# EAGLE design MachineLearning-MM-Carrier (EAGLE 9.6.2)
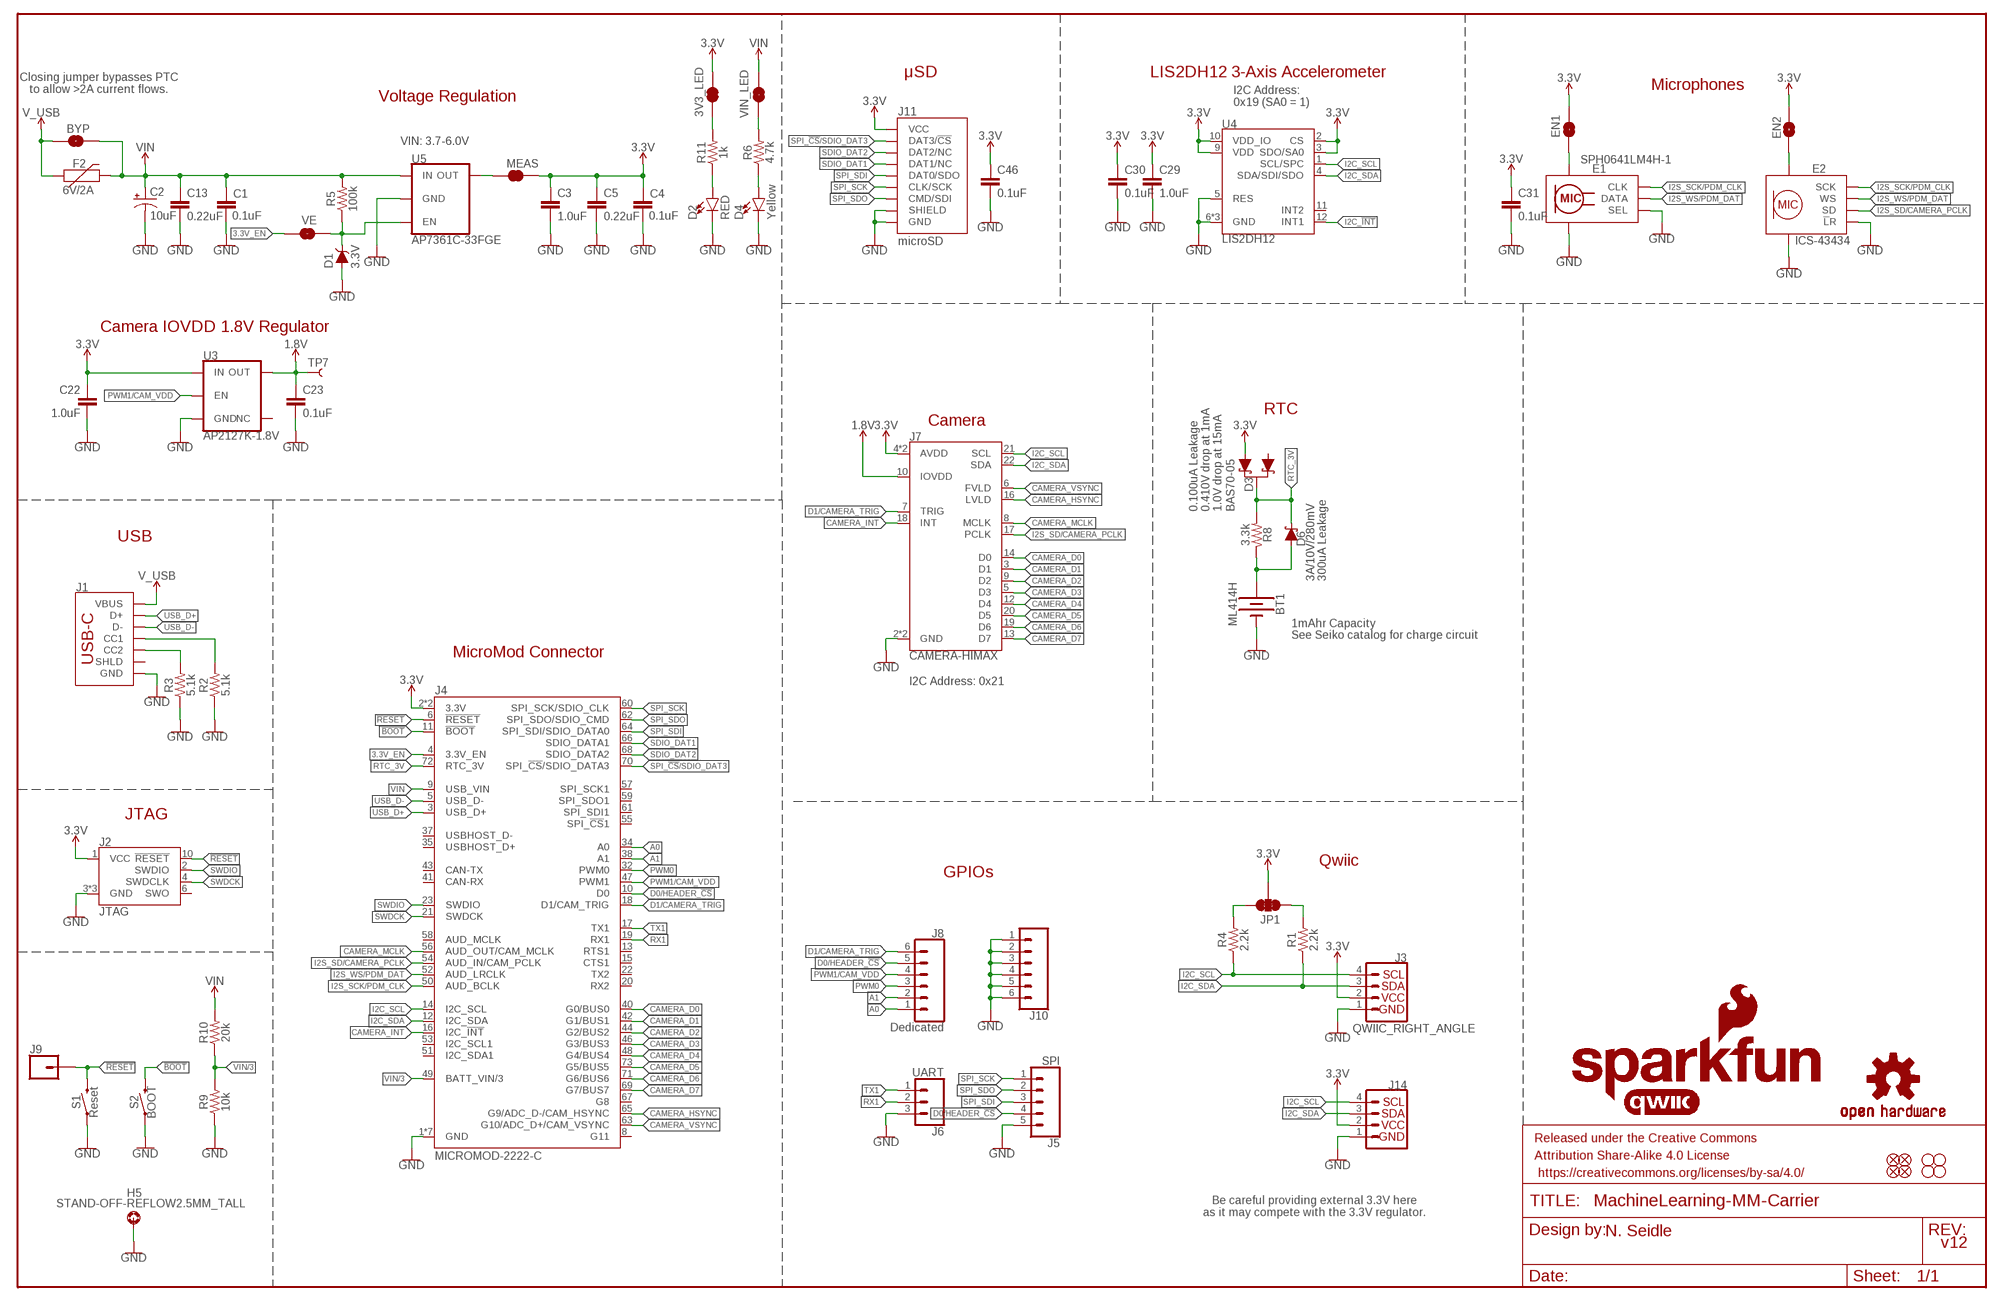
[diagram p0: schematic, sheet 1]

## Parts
3V3_LED  JUMPER-SMT_2_NC_TRACE_SILK  [SMT-JUMPER_2_NC_TRACE_SILK]
BT1  ML414H  ML414H_IV01E_BATTERY  [ML414H_IV01E]
BYP  JUMPER-SMT_2_NO_SILK  [SMT-JUMPER_2_NO_SILK]
C1  0.1uF  0.1UF-0603-25V-(+80/-20%)  [0603]
C2  10uF  10UF-POLAR-EIA3216-16V-10%(TANT)  [EIA3216]
C3  1.0uF  1.0UF-0603-16V-10%  [0603]
C4  0.1uF  0.1UF-0603-25V-(+80/-20%)  [0603]
C5  0.22uF  0.22UF-0603-25V-10%  [0603]
C13  0.22uF  0.22UF-0603-25V-10%  [0603]
C22  1.0uF  1.0UF-0603-16V-10%  [0603]
C23  0.1uF  0.1UF-0603-100V-10%  [0603]
C29  1.0uF  1.0UF-0603-16V-10%  [0603]
C30  0.1uF  0.1UF-0603-25V-(+80/-20%)  [0603]
C31  0.1uF  0.1UF-0603-25V-(+80/-20%)  [0603]
C46  0.1uF  0.1UF-0603-25V-(+80/-20%)  [0603]
D1  3.3V  DIODE-ZENER-MM3Z3V3T1G  [SOD-323]
D2  RED  LED-RED0603  [LED-0603]
D3  BAS70-05  DIODE-SCHOTTKY-DUAL  [SOT23-3]
D4  Yellow  LED-YELLOW0603  [LED-0603]
D6  3A/10V/280mV  DIODE-SCHOTTKY-BAT60A  [SOD-323]
E1  SPH0641LM4H-1  SPH0641LM4H-1_MICROPHONE  [SPH0641LM4H-1_MICROPHONE]
E2  ICS-43434  [ICS-43434]
EN1  JUMPER-SMT_2_NC_TRACE_SILK  [SMT-JUMPER_2_NC_TRACE_SILK]
EN2  JUMPER-SMT_2_NO_SILK  [SMT-JUMPER_2_NO_SILK]
F2  6V/2A  PPTC_6V2A  [1210]
FD1  FIDUCIALUFIDUCIAL  [FIDUCIAL-MICRO]
FD2  FIDUCIALUFIDUCIAL  [FIDUCIAL-MICRO]
FD3  FIDUCIALUFIDUCIAL  [FIDUCIAL-MICRO]
FD4  FIDUCIALUFIDUCIAL  [FIDUCIAL-MICRO]
FRAME1  FRAME-LEDGER  [CREATIVE_COMMONS]
H1  STAND-OFF  [STAND-OFF]
H2  STAND-OFF  [STAND-OFF]
H3  STAND-OFF  [STAND-OFF]
H4  STAND-OFF  [STAND-OFF]
H5  STAND-OFF-REFLOW2.5MM_TALL  [STAND-OFF-REFLOW-M2.5]
J1  USB_C_2-LAYER_PADS  [USB-C-16P-2LAYER-PADS]
J2  JTAG  CORTEX_JTAG_DEBUG_MINIMUM_PTH  [2X5-PTH-1.27MM]
J3  QWIIC_RIGHT_ANGLE  QWIIC_CONNECTORJS-1MM  [JST04_1MM_RA]
J4  MICROMOD-2222-C  [M.2-CONNECTOR-E]
J5  SPI  CONN_05NO_SILK  [1X05_NO_SILK]
J6  UART  CONN_031X03_NO_SILK  [1X03_NO_SILK]
J7  CAMERA-HIMAX  [FPC05024-42201]
J8  Dedicated  CONN_06NO_SILK_NO_POP  [1X06_NO_SILK]
J9  CONN_01PTH_NO_SILK_YES_STOP  [1X01_NO_SILK]
J10  CONN_06NO_SILK_NO_POP  [1X06_NO_SILK]
J11  microSD  MICRO-SD-SDIOPUSH-PUSH  [MICRO-SD-SOCKET]
J14  I2C_STANDARD_NO_SILK  [1X04_NO_SILK]
JP1  JUMPER-SMT_3_2-NC_TRACE_SILK  [SMT-JUMPER_3_2-NC_TRACE_SILK]
LOGO1  SFE_LOGO_NAME_FLAME.1_INCH  [SFE_LOGO_NAME_FLAME_.1]
LOGO2  QWIIC_LOGO_CONNECTOR  [QWIIC_5.5MM]
LOGO3  OSHW-LOGOMINI  [OSHW-LOGO-MINI]
MEAS  JUMPER-COMBO_2_NC_TRACE  [COMBO-JUMPER_2_NC_TRACE]
R1  2.2k  2.2KOHM-0603-1/10W-1%  [0603]
R2  5.1k  5.1KOHM5.1KOHM-0603-1/10W-1%  [0603]
R3  5.1k  5.1KOHM5.1KOHM-0603-1/10W-1%  [0603]
R4  2.2k  2.2KOHM-0603-1/10W-1%  [0603]
R5  100k  100KOHM-0603-1/10W-1%  [0603]
R6  4.7k  4.7KOHM-0603-1/10W-1%  [0603]
R8  3.3k  3.3KOHM-0603-1/10W-1%  [0603]
R9  10k  10KOHM-0603-1/10W-1%  [0603]
R10  20k  20KOHM-0603-1/10W-1%  [0603]
R11  1k  1KOHM-0603-1/10W-1%  [0603]
S1  Reset  MOMENTARY-SWITCH-SPST-SMD-5.2-TALL-REDUNDANT  [TACTILE_SWITCH_SMD_5.2MM]
S2  BOOT  MOMENTARY-SWITCH-SPST-SMD-5.2-TALL-REDUNDANT  [TACTILE_SWITCH_SMD_5.2MM]
TP7  TEST-POINT3X5  [PAD.03X.05]
U3  AP2127K-1.8V  V_REG_AP2127K-1.8V  [SOT23-5]
U4  LIS2DH12  [LGA-12-LISDH12]
U5  AP7361C-33FGE  AP7361C-33FGEUDFN-8  [UDFN-8]
VE  JUMPER-SMT_2_NO_SILK  [SMT-JUMPER_2_NO_SILK]
VIN_LED  JUMPER-SMT_2_NC_TRACE_SILK  [SMT-JUMPER_2_NC_TRACE_SILK]

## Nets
1.8V: C23.1 J7.10(IOVDD) TP7.P$1 U3.5(OUT)
3.3V: 3V3_LED.2 C3.1 C4.1 C5.1 C22.1 C29.1 C30.1 C31.1 C46.1 D3.2(A1) EN1.2 EN2.2 J2.1(VCC) J3.2 J4.2(3.3V) J4.74(3.3V) J7.4(AVDD) J7.11(AVDD) J11.VCC J14.2 JP1.2 MEAS.2 MEAS.4 U3.1(IN) U4.2(CS) U4.3(SDO/SA0) U4.9(VDD) U4.10(VDD_IO)
3.3V_EN: J4.4(3.3V_EN) VE.1
!BOOT!: J4.11(!BOOT!) S2.3 S2.4
!RESET!: J2.10(!RESET) J4.6(!RESET!) J9.1 S1.3 S1.4
A0: J4.34(A0) J8.1
A1: J4.38(A1) J8.2
CAMERA_D0: J4.40(G0/BUS0) J7.14(D0)
CAMERA_D1: J4.42(G1/BUS1) J7.3(D1)
CAMERA_D2: J4.44(G2/BUS2) J7.9(D2)
CAMERA_D3: J4.46(G3/BUS3) J7.5(D3)
CAMERA_D4: J4.48(G4/BUS4) J7.12(D4)
CAMERA_D5: J4.73(G5/BUS5) J7.20(D5)
CAMERA_D6: J4.71(G6/BUS6) J7.19(D6)
CAMERA_D7: J4.69(G7/BUS7) J7.13(D7)
CAMERA_HSYNC: J4.65(G9/ADC_D-/CAM_HSYNC) J7.16(LVLD)
CAMERA_INT: J4.16(I2C_!INT!) J7.18(INT)
CAMERA_MCLK: J4.56(AUD_OUT/CAM_MCLK) J7.8(MCLK)
CAMERA_VSYNC: J4.63(G10/ADC_D+/CAM_VSYNC) J7.6(FVLD)
D0/HEADER_!CS!: J4.10(D0) J5.4 J8.5
D1/CAMERA_TRIG: J4.18(D1/CAM_TRIG) J7.7(TRIG) J8.6
GND: BT1.- C1.2 C2.- C3.2 C4.2 C5.2 C13.2 C22.2 C23.2 C29.2 C30.2 C31.2 C46.2 D1.A D2.C D4.C E1.2(SEL) E1.3(GND) E1.6(GND) E1.7(GND) E1.8(GND) E2.2(!L!R) E2.3(GND) E2.7(GND) E2.8(GND) E2.9(GND) H5.1 J1.GND J1.GND2(GND) J2.3(GND) J2.5(GND) J2.9(GND) J3.1 J4.1(GND) J4.7(GND) J4.33(GND) J4.36(GND) J4.39(GND) J4.45(GND) J4.75(GND) J5.5 J6.3 J7.2(GND) J7.15(GND) J10.1 J10.2 J10.3 J10.4 J10.5 J10.6 J11.CD1(SHIELD) J11.GND J11.GND1(GND) J11.GND3(GND) J14.1 R2.1 R3.1 R9.1 S1.1 S1.2 S2.1 S2.2 U3.2(GND) U4.5(RES) U4.6(GND) U4.7(GND) U4.8(GND) U5.4(GND) U5.EP(GND)
I2C_!INT!: U4.12(INT1)
I2C_SCL: J3.4 J4.14(I2C_SCL) J7.21(SCL) J14.4 R4.1 U4.1(SCL/SPC)
I2C_SDA: J3.3 J4.12(I2C_SDA) J7.22(SDA) J14.3 R1.1 U4.4(SDA/SDI/SDO)
I2S_SCK/PDM_CLK: E1.4(CLK) E2.4(SCK) J4.50(AUD_BCLK)
I2S_SD/CAMERA_PCLK: E2.6(SD) J4.54(AUD_IN/CAM_PCLK) J7.17(PCLK)
I2S_WS/PDM_DAT: E1.1(DATA) E2.1(WS) J4.52(AUD_LRCLK)
N$1: R6.2 VIN_LED.1
N$2: JP1.3 R4.2
N$3: JP1.1 R1.2
N$4: E1.5(VDD) EN1.1
N$5: E2.5(VDD) EN2.1
N$6: 3V3_LED.1 R11.2
N$7: D2.A R11.1
N$8: D4.A R6.1
N$10: J1.A5(CC1) R2.2
N$11: J1.B5(CC2) R3.2
N$12: D1.C R5.1 U5.5(EN) VE.2
N$14: BT1.+ D6.A R8.1
PWM0: J4.32(PWM0) J8.3
PWM1/CAM_VDD: J4.47(PWM1) J8.4 U3.3(EN)
RTC_3V: D3.3(C) D6.C J4.72(RTC_3V) R8.2
RX1: J4.19(RX1) J6.2
SDIO_DAT1: J4.66(SDIO_DATA1) J11.DAT1(DAT1/NC)
SDIO_DAT2: J4.68(SDIO_DATA2) J11.DAT2(DAT2/NC)
SPI_!CS!/SDIO_DAT3: J4.70(SPI_!CS!/SDIO_DATA3) J11.CS/DAT3(DAT3/!CS!)
SPI_SCK: J4.60(SPI_SCK/SDIO_CLK) J5.1 J11.SCLK(CLK/SCK)
SPI_SDI: J4.64(SPI_SDI/SDIO_DATA0) J5.3 J11.DO/DAT0(DAT0/SDO)
SPI_SDO: J4.62(SPI_SDO/SDIO_CMD) J5.2 J11.DI/CMD(CMD/SDI)
SWDCK: J2.4(SWDCLK) J4.21(SWDCK)
SWDIO: J2.2(SWDIO) J4.23(SWDIO)
TX1: J4.17(TX1) J6.1
USB_D+: J1.A6(D+) J1.B6(D+) J4.3(USB_D+)
USB_D-: J1.A7(D-) J1.B7(D-) J4.5(USB_D-)
V_USB: BYP.1 F2.1 J1.VBUS1(VBUS) J1.VBUS2(VBUS)
VIN: BYP.2 C1.1 C2.+ C13.1 F2.2 J4.9(USB_VIN) R5.2 R10.2 U5.8(IN) VIN_LED.2
VIN/3: J4.49(BATT_VIN/3) R9.2 R10.1
VREG_3.3V: MEAS.1 MEAS.3 U5.1(OUT)
Unconnected: D3.1(A) J1.SHLD1(SHLD) J1.SHLD2(SHLD) J1.SHLD3(SHLD) J1.SHLD4(SHLD) J2.6(SWO) J4.8(G11) J4.13(RTS1) J4.15(CTS1) J4.20(RX2) J4.22(TX2) J4.35(USBHOST_D+) J4.37(USBHOST_D-) J4.41(CAN-RX) J4.43(CAN-TX) J4.51(I2C_SDA1) J4.53(I2C_SCL1) J4.55(SPI_!CS!1) J4.57(SPI_SCK1) J4.58(AUD_MCLK) J4.59(SPI_SDO1) J4.61(SPI_SDI1) J4.67(G8) J7.MNT1 J7.MNT2 U3.4(NC) U4.11(INT2)

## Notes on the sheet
- μSD | LIS2DH12 3-Axis Accelerometer
- Closing jumper bypasses PTC
  to allow >2A current flows.
- Microphones
- Voltage Regulation
- I2C Address:
  0x19 (SA0 = 1)
- VIN: 3.7-6.0V
- Camera IOVDD 1.8V Regulator
- RTC
- Camera
- 0.100uA Leakage
  0.410V drop at 1mA
  1.0V drop at 15mA
- USB
- 300uA Leakage
- 1mAhr Capacity
- See Seiko catalog for charge circuit
- MicroMod Connector
- I2C Address: 0x21
- JTAG
- Qwiic
- GPIOs
- Be careful providing external 3.3V here
  as it may compete with the 3.3V regulator.
- N. Seidle
- v12

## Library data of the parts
3V3_LED EN1 VIN_LED = SparkFun-Jumpers:JUMPER-SMT_2_NC_TRACE: Normally closed trace jumper
BT1 = SparkFun-Batteries:ML414H_IV01E_BATTERY: SEIKO ML414H-IV01E Reflowable Lithium Battery; PROD_ID: BATT-14267
BYP EN2 VE = SparkFun-Jumpers:JUMPER-SMT_2_NO: Normally open jumper
C1 C4 C30 C31 C46 = SparkFun-Capacitors:0.1UF: 0.1µF ceramic capacitors; PROD_ID: CAP-00810
C2 = SparkFun-Capacitors:10UF-POLAR: 10.0µF polarized capacitors; PROD_ID: CAP-00811
C3 C22 C29 = SparkFun-Capacitors:1.0UF: 1µF ceramic capacitors; PROD_ID: CAP-00868
C5 C13 = SparkFun-Capacitors:0.22UF: 0.22µF ceramic capacitors; PROD_ID: CAP-07822
C23 = SparkFun-Capacitors:0.1UF: 0.1µF ceramic capacitors; PROD_ID: CAP-08390
D1 = SparkFun-DiscreteSemi:DIODE-ZENER: Zener Diode; PROD_ID: DIO-11284
D2 = SparkFun-LED:LED-RED: Red SMD LED; PROD_ID: DIO-00819
D3 = SparkFun-DiscreteSemi:DIODE-SCHOTTKY-DUAL: Diodes Incorporated - BAS70-05 Dual Schottky Diode Two Schottky Diodes in a single SOT-23 package. Low reverse current (100 nA) Vf: Datasheet referenced for footprint; PROD_ID: DIO-14829
D4 = SparkFun-LED:LED-YELLOW: Yellow SMD LED; PROD_ID: DIO-09003
D6 = SparkFun-DiscreteSemi:DIODE-SCHOTTKY: Schottky diode; PROD_ID: DIO-14072
E1 = SparkFun-Sensors:SPH0641LM4H-1_MICROPHONE: SPH0641LM4H-1 Microphone A miniature, high-performance, low power, bottom port silicon digital microphone with a single bit PDM output.; PROD_ID: IC-14361
E2 = Teensy:ICS-43434; PROD_ID: COMP-14898
F2 = SparkFun-Fuses:PPTC: Resettable Fuse PPTC; PROD_ID: RES-14313
FD1-FD4 = SparkFun-Aesthetics:FIDUCIAL: Fiducial Alignment Points
FRAME1 = SparkFun-Aesthetics:FRAME-LEDGER: Schematic Frame - Ledger
H1-H4 = SparkFun-Hardware:STAND-OFF: Stand Off
H5 = SparkFun-Hardware:STAND-OFF-REFLOW: Stand Off Reflow Compatible; PROD_ID: HW-14899
J1 = SparkFun-Connectors:USB_C: USB Type C 16Pin Connector Super Speed pins not available on the 16-pin purely SMD connector so this part is best for USB 2.0 implementations. D1 and D2 are tied together enabling D+/- no matter which way the cable is plugged into the connector. The two channel configuration pins (CC1/2) are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; PROD_ID: CONN-14122
J2 = SparkFun-Connectors:CORTEX_JTAG_DEBUG_MINIMUM: Cortex Debug Connector - 10 pin Supports JTAG debug, Serial Wire debug, and Serial Wire Viewer. PTH and SMD connector options available. General Connector Information Products: PTH Connector -via Digi-Key SparkFun PSoc SparkFun T
J3 = SparkFun-Connectors:QWIIC_CONNECTOR: SparkFun I2C Standard Qwiic Connector An SMD 1mm pitch JST connector makes it easy and quick (get it? Qwiic?) to connect I2C devices to each other. The Qwiic system enables fast and solderless connection between popular platforms and various sensors and actuators. We carry 200mm, 100mm, 50mm, and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; PROD_ID: CONN-13694
J4 = SparkFun-MicroMod:MICROMOD: MicroMod Connector Description: A card edge connector and mating PCB connector to allow various MicroMod Processor Boards to be coupled with various carrier boards of different capabilities. Based on the M.2 standard.; PROD_ID: CONN-14877
J5 = SparkFun-Connectors:CONN_05: Multi connection point. Often used as Generic Header-pin footprint for 0.1 inch spaced/style header connections On any of the 0.1 inch spaced packages, you can populate with these: Break Away Headers - Straight (PRT-00116) Break Away Male Headers - Right Angle (PRT-00553) Female Headers (PRT-00115)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
J6 = SparkFun-Connectors:CONN_03: Multi connection point. Often used as Generic Header-pin footprint for 0.1 inch spaced/style header connections On any of the 0.1 inch spaced packages, you can populate with these: Break Away Headers - Straight (PRT-00116) Break Away Male Headers - Right Angle (PRT-00553) Female Headers (PRT-00115)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
J7 = SparkFun-Connectors:CAMERA-HIMAX
J8 J10 = SparkFun-Connectors:CONN_06: Multi connection point. Often used as Generic Header-pin footprint for 0.1 inch spaced/style header connections On any of the 0.1 inch spaced packages, you can populate with these: Break Away Headers - Straight (PRT-00116) Break Away Male Headers - Right Angle (PRT-00553) Female Headers (PRT-00115)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
J9 = SparkFun-Connectors:CONN_01: Single connection point. Often used as Generic Header-pin footprint for 0.1 inch spaced/style header connections
J11 = SparkFun-Connectors:MICRO-SD-SDIO: microSD Socket for Transflash Push-push type µSD socket. tDoc lines correctly indicate media card edge positions when inserting (unlocked, locked, depressed). NOTE: CD1 and CD2 are connected internally, and the default detect state of the socket is detect pin to ground. SparkFun Products: WAV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; PROD_ID: CONN-07820
J14 = SparkFun-Connectors:I2C_STANDARD: SparkFun I2C Standard Pinout Header SparkFun has standardized on a pinout for all I2C based sensor breakouts. This pinout allows I2C boards to be plugged directly into the headers on Arduino Uno compatible boards, and to be daisy chained easily. Example SparkFun Products: SparkFun Atmospheric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
JP1 = SparkFun-Jumpers:JUMPER-SMT_3_2-NC_TRACE: Normally closed trace jumper (2 of 2 connections) This jumper has a trace between all three pads so they are normally closed (NC). Use a razor knife to open the connection(s). For best results follow the IPC guidelines for cutting traces: Cutout at least 0.063 mm (0.005 in). Remove all loose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
LOGO1 = SparkFun-Aesthetics:SFE_LOGO_NAME_FLAME: SparkFun Font Logo w/ Flame
LOGO2 = SparkFun-Aesthetics:QWIIC_LOGO: Qwiic Logos for placement on schematic and PCB. The 5.5mm silk logo is best for placing next to Qwiic connector.
LOGO3 = SparkFun-Aesthetics:OSHW-LOGO: Open-Source Hardware (OSHW) Logo
MEAS = SparkFun-Jumpers:JUMPER-COMBO_2_NC_TRACE
R1 R4 = SparkFun-Resistors:2.2KOHM: 2.2kΩ resistor; PROD_ID: RES-08272
R2 R3 = SparkFun-Resistors:5.1KOHM; PROD_ID: RES-12083
R5 = SparkFun-Resistors:100KOHM: 100kΩ resistor; PROD_ID: RES-07828
R6 = SparkFun-Resistors:4.7KOHM: 4.7kΩ resistor; PROD_ID: RES-07857
R8 = SparkFun-Resistors:3.3KOHM: 3.3kΩ resistor; PROD_ID: RES-07851
R9 = SparkFun-Resistors:10KOHM: 10kΩ resistor; PROD_ID: RES-00824
R10 = SparkFun-Resistors:20KOHM: 20kΩ resistor; PROD_ID: RES-09383
R11 = SparkFun-Resistors:1KOHM: 1kΩ resistor; PROD_ID: RES-07856
S1 S2 = SparkFun-Switches:MOMENTARY-SWITCH-SPST: Momentary Switch (Pushbutton) - SPST; PROD_ID: SWCH-14139
TP7 = SparkFun-Connectors:TEST-POINT: SparkFun Test Points
U3 = SparkFun-IC-Power:V_REG_AP2127: AP2127 - 300mA CMOS LDO Regulator w/ Enable The AP2127 is CMOS process low dropout linear regulator with enable function, the regulator delivers a guaranteed 300mA (min.) continuous load current. Features Output Voltage Accuracy: ±1.5% Output Current: 300mA (Min.) Foldback Short Current Protection: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; PROD_ID: VREG-14239
U4 = SparkFun-Sensors:LIS2DH12; DIGIKEY: 497-14851-2-ND; PROD_ID: IC-14229
U5 = SparkFun-IC-Power:AP7361C-33FGE: AP7361C 3.3V LDO Regulator; PROD_ID: VREG-14094

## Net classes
0 default: width 0 mm, drill 0 mm
1 power: width 0.762 mm

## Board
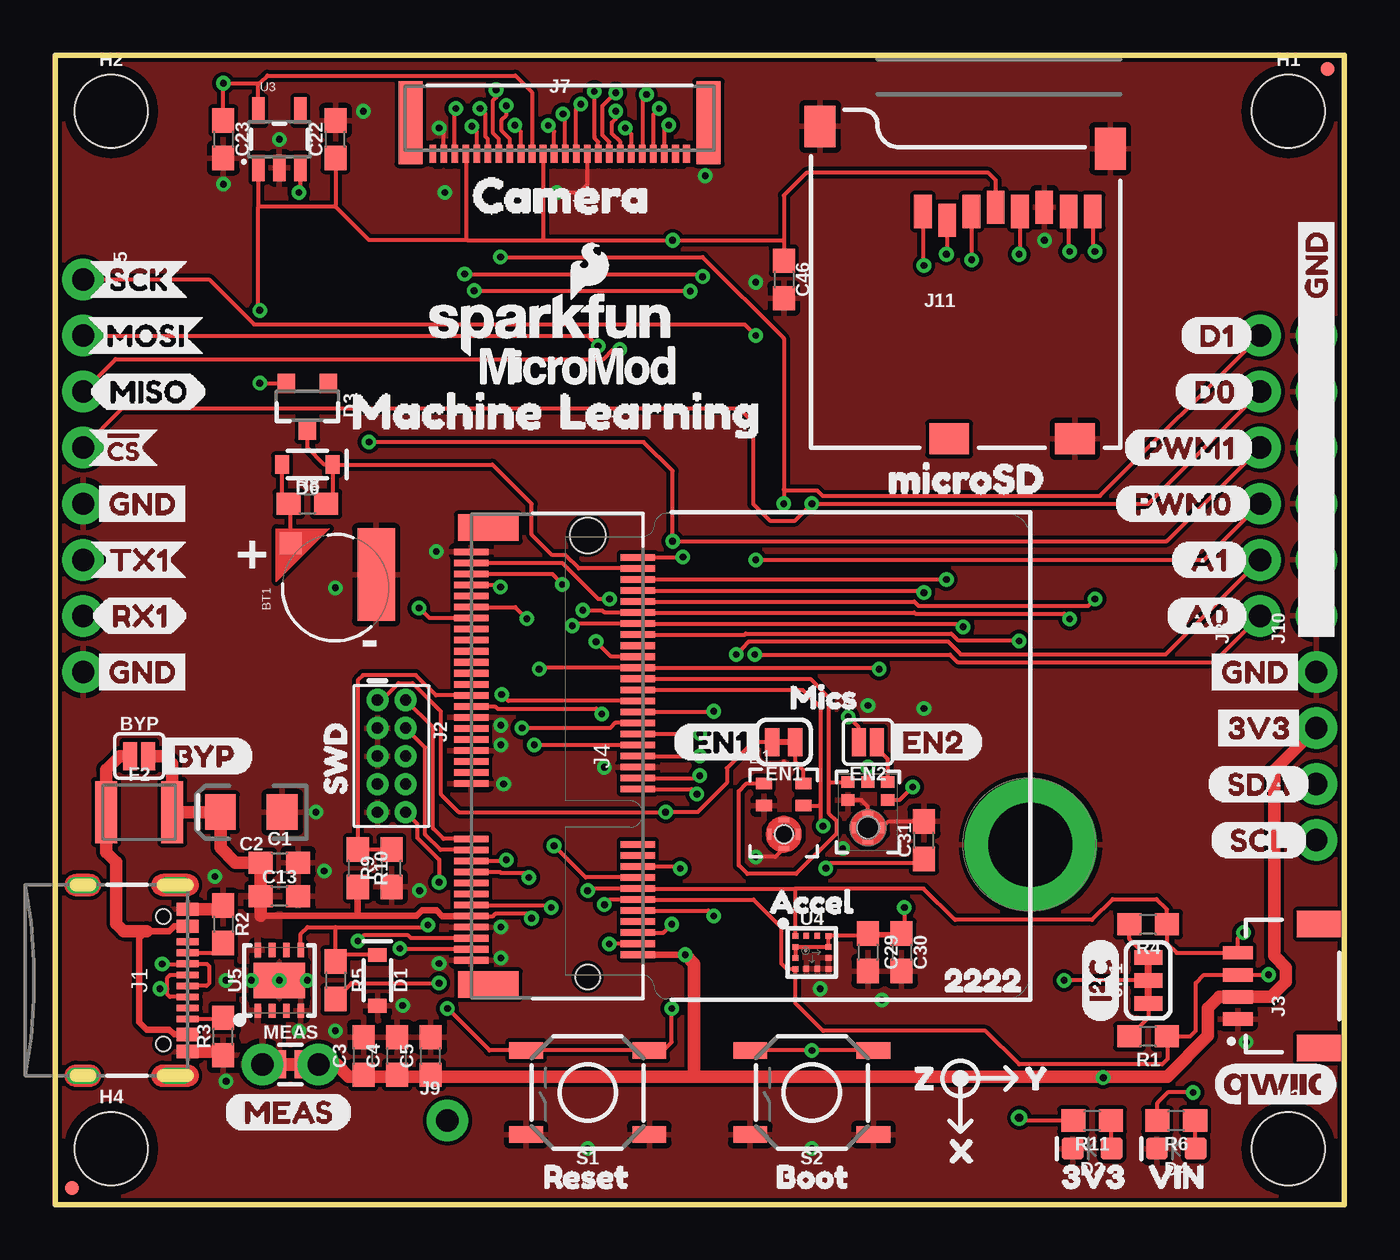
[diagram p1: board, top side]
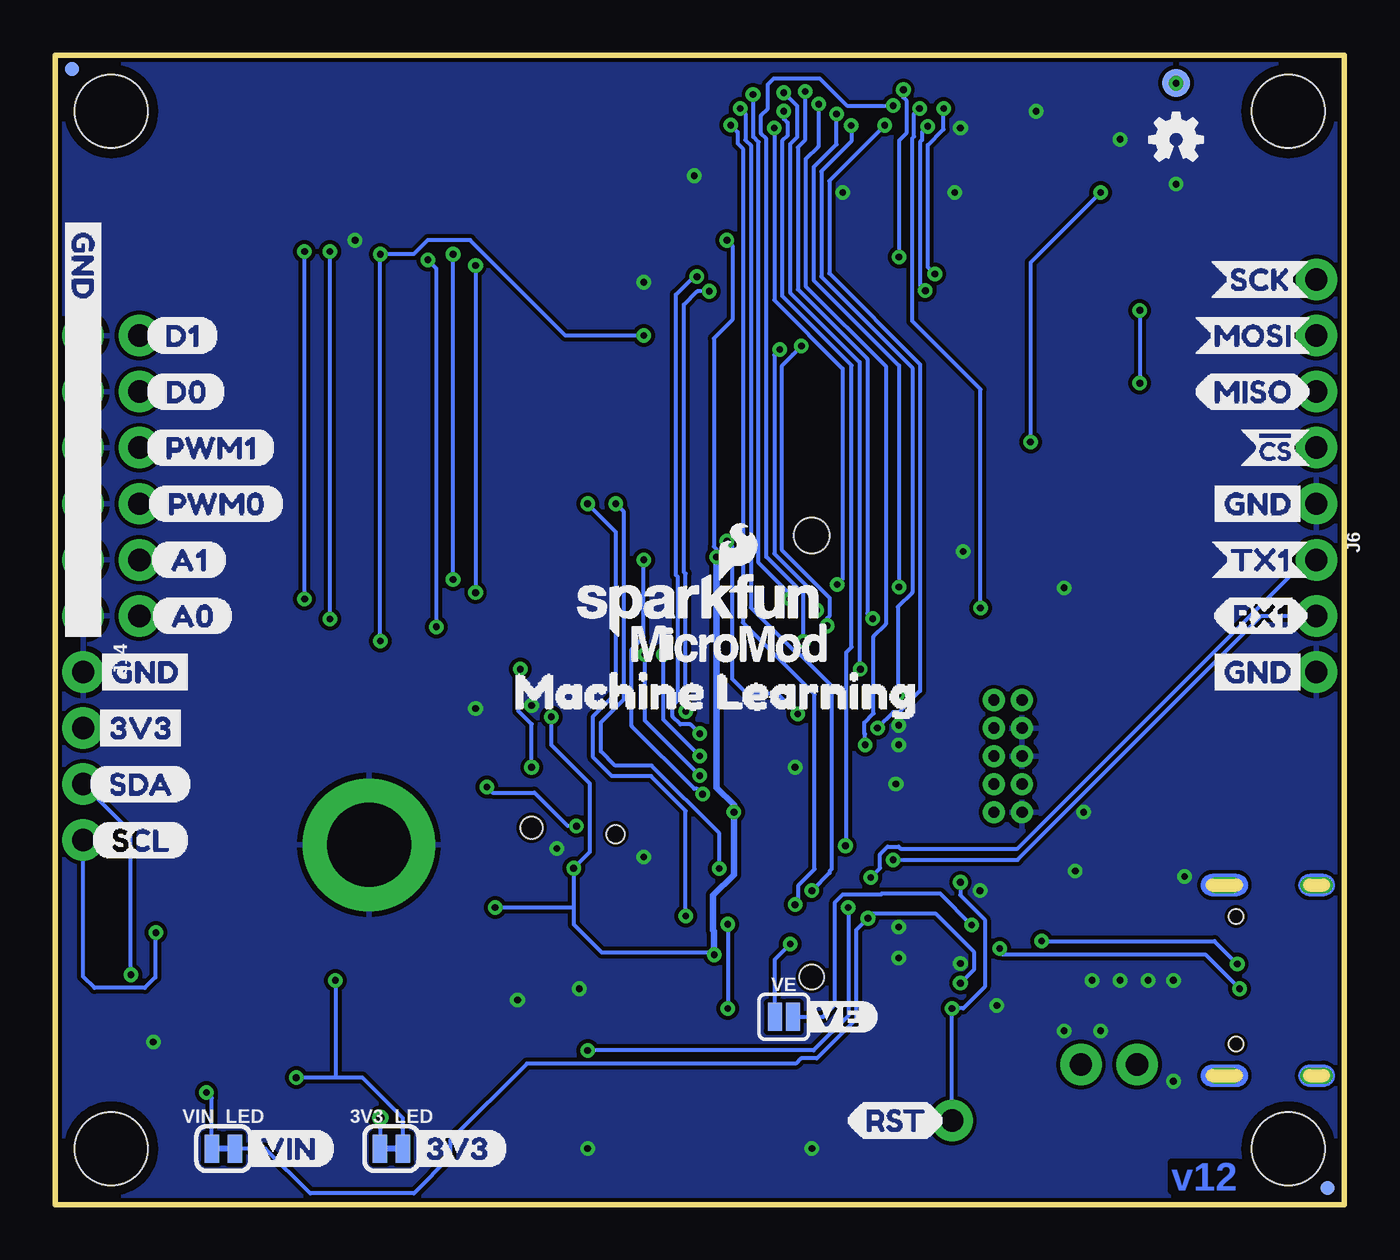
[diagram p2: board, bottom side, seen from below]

Size 58.42 x 52.07 mm. Coordinates in mm from the lower left corner, seen from the top.
Outline: 0,0 0,52.07 58.42,52.07 58.42,0 0,0
Copper layers (1*16): Top 0.035mm / dielectric 1.5mm / Bottom 0.035mm
Design rules "SparkFun-2-layer-TIGHT *": minimum track width 7mil, minimum drill 12mil, track to track 7mil, track to pad 7mil, pad to pad 7mil, via to via 7mil, smd to smd 7mil, copper to edge 7mil, drill to drill 7mil, minimum pad ring 7mil, minimum via ring 7mil, stop-mask expansion 4mil, vias tented up to drill 25mil, thermal gap 10mil

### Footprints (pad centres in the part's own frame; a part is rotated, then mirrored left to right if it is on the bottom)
SMT-JUMPER_2_NC_TRACE_SILK = smd 0.66 x 1.27: 1 -0.521,0; 2 0.521,0
ML414H_IV01E = smd 1 x 1: + 2.022,2.032 | smd 4.2 x 1.7: - 0.6,-1.85
SMT-JUMPER_2_NO_SILK = smd 0.635 x 1.27: 1 -0.406,0; 2 0.406,0
0603 = smd 1.1 x 1: 1 -0.85,0; 2 0.85,0
EIA3216 = smd 1.4 x 1.6: + 1.4,0; - -1.4,0
SOD-323 = smd 0.63 x 0.83: A 1.15,0; C -1.15,0
LED-0603 = smd 1 x 1: A -0.877,0; C 0.877,0
SOT23-3 = smd 0.8 x 0.9: 1 -0.95,-1; 2 0.95,-1; 3 0,1.1
SPH0641LM4H-1_MICROPHONE = smd 0.725 x 0.522: 1 -0.9,1.3; 2 -0.9,0.3; 4 0.9,0.3; 5 0.9,1.3 | smd 0.5 x 0.2: 3 0,-1.65; 8 0,-0.35 | smd 0.2 x 0.5: 6 -0.65,-1; 7 0.65,-1 | hole 0.8: 0,-1
ICS-43434 = smd 0.522 x 0.6: 1 -1.364,-0.9; 2 -0.542,-0.9; 4 -0.542,0.9; 5 -1.364,0.9; 6 -1.364,0 | smd 0.2 x 0.5: 3 1.36,0; 8 0.06,0 | smd 0.5 x 0.2: 7 0.71,0.65; 9 0.71,-0.65 | hole 1: 0.71,0
1210 = smd 1 x 2.8: 1 -1.5,0; 2 1.5,0
FIDUCIAL-MICRO = smd 0.635 x 0.635: 1 0,0
STAND-OFF = hole 3.302: 0,0
STAND-OFF-REFLOW-M2.5 = drill 3.8 pad 6: 1 0,0
USB-C-16P-2LAYER-PADS = smd 0.3 x 1: A5 -1.25,-0.34; A6 -0.25,-0.34; A7 0.25,-0.34; A8 1.25,-0.34; B5 1.75,-0.34; B6 0.75,-0.34; B7 -0.75,-0.34; B8 -1.75,-0.34 | smd 0.6 x 1: GND -3.225,-0.34; GND2 3.225,-0.34; VBUS1 -2.45,-0.34; VBUS2 2.45,-0.34 | drill 0.4 pad 0.6 long: SHLD1 -4.318,-0.915; SHLD2 4.318,-0.915; SHLD3 -4.318,-5.095; SHLD4 4.318,-5.095 | hole 0.65: -2.89,-1.445; 2.89,-1.445
2X5-PTH-1.27MM = drill 0.508 pad 1: 1 -2.54,-0.635; 2 -2.54,0.635; 3 -1.27,-0.635; 4 -1.27,0.635; 5 0,-0.635; 6 0,0.635; 7 1.27,-0.635; 8 1.27,0.635; 9 2.54,-0.635; 10 2.54,0.635
JST04_1MM_RA = smd 0.6 x 1.35: 1 -1.5,0; 2 -0.5,0; 3 0.5,0; 4 1.5,0 | smd 1.2 x 2: NC1 2.8,-3.675; NC2 -2.8,-3.675
M.2-CONNECTOR-E = smd 0.3 x 1.55: 1 9.25,-5.275; 2 9,2.275; 3 8.75,-5.275; 4 8.5,2.275; 5 8.25,-5.275; 6 8,2.275; 7 7.75,-5.275; 8 7.5,2.275; 9 7.25,-5.275; 10 7,2.275; 11 6.75,-5.275; 12 6.5,2.275; 13 6.25,-5.275; 14 6,2.275; 15 5.75,-5.275; 16 5.5,2.275; 17 5.25,-5.275; 18 5,2.275; 19 4.75,-5.275; 20 4.5,2.275; 21 4.25,-5.275; 22 4,2.275; 23 3.75,-5.275; 32 1.5,2.275; 33 1.25,-5.275; 34 1,2.275; 35 0.75,-5.275; 36 0.5,2.275; 37 0.25,-5.275; 38 0,2.275; 39 -0.25,-5.275; 40 -0.5,2.275; 41 -0.75,-5.275; 42 -1,2.275; 43 -1.25,-5.275; 44 -1.5,2.275; 45 -1.75,-5.275; 46 -2,2.275; 47 -2.25,-5.275; 48 -2.5,2.275; 49 -2.75,-5.275; 50 -3,2.275; 51 -3.25,-5.275; 52 -3.5,2.275; 53 -3.75,-5.275; 54 -4,2.275; 55 -4.25,-5.275; 56 -4.5,2.275; 57 -4.75,-5.275; 58 -5,2.275; 59 -5.25,-5.275; 60 -5.5,2.275; 61 -5.75,-5.275; 62 -6,2.275; 63 -6.25,-5.275; 64 -6.5,2.275; 65 -6.75,-5.275; 66 -7,2.275; 67 -7.25,-5.275; 68 -7.5,2.275; 69 -7.75,-5.275; 70 -8,2.275; 71 -8.25,-5.275; 72 -8.5,2.275; 73 -8.75,-5.275; 74 -9,2.275; 75 -9.25,-5.275 | smd 1.2 x 2.75: A1 10.35,-4.5; A2 -10.35,-4.5 | hole 1.1: 10,0 | hole 1.6: -10,0
1X05_NO_SILK = drill 1.016 pad 1.88: 1 0,0; 2 2.54,0; 3 5.08,0; 4 7.62,0; 5 10.16,0
1X03_NO_SILK = drill 1.016 pad 1.88: 1 0,0; 2 2.54,0; 3 5.08,0
FPC05024-42201 = smd 0.3 x 0.8: 1 5.75,0.4; 2 5.25,0.4; 3 4.75,0.4; 4 4.25,0.4; 5 3.75,0.4; 6 3.25,0.4; 7 2.75,0.4; 8 2.25,0.4; 9 1.75,0.4; 10 1.25,0.4; 11 0.75,0.4; 12 0.25,0.4; 13 -0.25,0.4; 14 -0.75,0.4; 15 -1.25,0.4; 16 -1.75,0.4; 17 -2.25,0.4; 18 -2.75,0.4; 19 -3.25,0.4; 20 -3.75,0.4; 21 -4.25,0.4; 22 -4.75,0.4; 23 -5.25,0.4; 24 -5.75,0.4 | smd 1.1 x 3.75: MNT1 -6.75,-1; MNT2 6.75,-1
1X06_NO_SILK = drill 1.016 pad 1.88: 1 0,0; 2 2.54,0; 3 5.08,0; 4 7.62,0; 5 10.16,0; 6 12.7,0
1X01_NO_SILK = drill 1.016 pad 1.88: 1 0,0
MICRO-SD-SOCKET = smd 1.8 x 1.4: CD1 -2.05,0.4; CD2 -7.75,0.4 | smd 0.8 x 1.5: CS/DAT3 -7.84,10.3; DAT1 -1.24,10.7; DAT2 -8.94,10.7; DI/CMD -6.74,10.7; DO/DAT0 -2.34,10.7; GND -3.44,10.9; SCLK -4.54,10.7; VCC -5.64,10.9 | smd 1.4 x 1.9: GND1 -13.6,14.55; GND3 -0.45,13.55
1X04_NO_SILK = drill 1.016 pad 1.88: 1 0,0; 2 2.54,0; 3 5.08,0; 4 7.62,0
SMT-JUMPER_3_2-NC_TRACE_SILK = smd 0.66 x 1.27: 1 -1.041,0; 2 0,0; 3 1.041,0
COMBO-JUMPER_2_NC_TRACE = smd 0.635 x 1.27: 1 -0.508,0; 2 0.508,0 | drill 1.016 pad 1.88: 3 -1.27,0; 4 1.27,0
TACTILE_SWITCH_SMD_5.2MM = smd 1.524 x 0.762: 1 -2.794,1.905; 2 2.794,1.905; 3 -2.794,-1.905; 4 2.794,-1.905
PAD.03X.05 = smd 1.27 x 1.27: P$1 0,0
SOT23-5 = smd 0.55 x 1.2: 1 -0.95,-1.3; 2 0,-1.3; 3 0.95,-1.3; 4 0.95,1.3; 5 -0.95,1.3
LGA-12-LISDH12 = smd 0.275 x 0.25: 1 -0.75,0.75; 2 -0.75,0.25; 3 -0.75,-0.25; 4 -0.75,-0.75; 7 0.75,-0.75; 8 0.75,-0.25; 9 0.75,0.25; 10 0.75,0.75 | smd 0.25 x 0.275: 5 -0.25,-0.75; 6 0.25,-0.75; 11 0.25,0.75; 12 -0.25,0.75
UDFN-8 = smd 0.3 x 0.65: 1 -0.975,-1.375; 2 -0.325,-1.375; 3 0.325,-1.375; 4 0.975,-1.375; 5 0.975,1.375; 6 0.325,1.375; 7 -0.325,1.375; 8 -0.975,1.375 | smd 2.35 x 1.6: EP 0,0

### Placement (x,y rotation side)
3V3_LED  43.18,2.54 0 bottom
BT1  12.7,27.94 90 top
BYP  3.81,20.32 0 top
C1  10.16,15.49 0 top
C2  8.89,17.78 180 top
C3  13.97,6.73 90 top
C4  15.49,6.73 90 top
C5  17.02,6.73 90 top
C13  10.16,13.97 0 top
C22  12.7,48.26 90 top
C23  7.62,48.26 270 top
C29  36.83,11.43 270 top
C30  38.35,11.43 270 top
C31  39.37,16.51 90 top
C46  33.02,41.91 270 top
D1  14.61,10.16 270 top
D2  46.99,2.54 180 top
D3  11.43,36.2 180 top
D4  50.8,2.54 180 top
D6  11.43,33.53 180 top
E1  33.02,17.78 0 top
E2  36.83,17.78 270 top
EN1  33.02,20.95 180 top
EN2  36.83,20.95 180 top
F2  3.81,17.78 0 top
FD1  0.76,0.76 0 top
FD2  57.66,51.44 0 top
FD3  0.76,0.76 0 bottom
FD4  57.66,51.44 0 bottom
FRAME1  not placed on the board
H1  55.88,49.53 0 top
H2  2.54,49.53 0 top
H3  55.88,2.54 0 top
H4  2.54,2.54 0 top
H5  44.2,16.3 0 top
J1  6.35,10.16 270 top
J2  15.24,20.32 270 top
J3  53.59,9.91 90 top
J4  24.13,20.32 270 top
J5  1.27,41.91 270 top
J6  1.27,29.21 270 bottom
J7  22.86,48.01 180 top
J8  54.61,26.67 90 top
J9  17.78,3.81 0 top
J10  57.15,26.67 90 top
J11  48.26,34.29 0 top
J14  57.15,24.13 270 bottom
JP1  49.53,10.16 90 top
LOGO1  22.48,39.88 0 top
LOGO2  55.31,5.46 0 top
LOGO3  7.62,48.26 0 bottom
LOGO4  SFE_LOGO_NAME_FLAME.1_INCH  [SFE_LOGO_NAME_FLAME_.1]  29.21,27.18 0 bottom
MEAS  10.67,6.35 0 top
R1  49.53,7.62 180 top
R2  7.62,12.7 270 top
R3  7.62,7.62 90 top
R4  49.53,12.7 180 top
R5  12.7,10.16 270 top
R6  50.8,3.81 180 top
R8  11.43,31.75 0 top
R9  15.24,15.24 90 top
R10  13.72,15.24 270 top
R11  46.99,3.81 180 top
S1  24.13,5.08 180 top
S2  34.29,5.08 180 top
TP7  7.62,50.8 0 bottom
U3  10.16,48.26 0 top
U4  34.29,11.43 0 top
U5  10.16,10.16 0 top
U$1  [ACCEL6]  31.5,13.72 0 top
U$2  [RESET3]  21.21,1.27 0 top
U$3  [CAMERA5]  17.53,45.72 0 top
U$4  [LEARNING3]  21.46,35.94 0 top
U$5  [MEAS]  7.62,4.19 0 top
U$6  [GND_P]  1.52,31.75 0 top
U$7  [MOSI_O]  1.4,39.37 0 top
U$8  [MISO_I]  1.52,36.83 0 top
U$9  [SCK_O]  1.52,41.91 0 top
U$10  [!CS_O]  1.27,34.29 0 top
U$11  [GND_P]  57.15,40.13 90 top
U$12  [D13]  50.93,39.37 0 top
U$13  [D13]  54.36,39.37 0 bottom
U$14  [D02]  50.67,36.83 0 top
U$15  [PWM10]  48.39,34.29 0 top
U$16  [D02]  54.36,36.83 0 bottom
U$17  [SWD3]  12.7,17.65 90 top
U$18  [RST_I]  22.61,3.81 0 bottom
U$19  [BOOT2]  31.75,1.27 0 top
U$20  [3V31]  42.55,2.54 0 bottom
U$21  [3V3_TO]  44.7,1.27 0 top
U$22  [MACHINE2]  12.06,35.94 0 top
U$23  [VIN_TO]  48.64,1.27 0 top
U$24  [MICROMOD_LOGO_.35]  23.62,37.97 0 top
U$25  [RX10]  1.65,26.67 0 top
U$26  [MICS0]  32.38,22.99 0 top
U$27  [EN13]  27.94,20.95 0 top
U$28  [VIN0]  50.04,2.54 0 bottom
U$29  [RX10]  5.97,26.67 0 bottom
U$30  [MICROSD_TO_50]  36.58,32.89 0 top
U$31  [TX13]  6.1,29.21 0 bottom
U$32  [GND_P]  6.35,24.13 0 bottom
U$33  [BYP0]  4.45,20.32 0 top
U$34  [MICROMOD_LOGO_.35]  27.94,25.4 0 bottom
U$36  [GND_P]  56.77,24.13 0 bottom
U$37  [I2C]  47.37,8.26 90 top
U$38  [3V3_P]  56.9,21.59 0 bottom
U$39  [SDA_IO]  56.9,19.05 0 bottom
U$40  [SCL_IO]  56.77,16.51 0 bottom
U$41  [TX13]  1.52,29.21 0 top
U$42  [GND_P]  1.52,24.13 0 top
U$43  [A00]  50.29,26.67 0 top
U$44  [A00]  54.1,26.67 0 bottom
U$45  [GND_P]  51.94,24.13 0 top
U$46  [3V3_P]  52.2,21.59 0 top
U$47  [SDA_IO]  52.2,19.05 0 top
U$48  [SCL_IO]  52.32,16.51 0 top
U$49  [SCK_O]  6.1,41.91 0 bottom
U$50  [MOSI_O]  6.86,39.37 0 bottom
U$51  [MISO_I]  6.86,36.83 0 bottom
U$52  [!CS_O]  4.95,34.29 0 bottom
U$53  [GND_P]  6.35,31.75 0 bottom
U$54  [GND_P]  57.15,44.96 270 bottom
U$55  [22229]  39.37,10.16 0 top
U$56  [X0]  39.62,2.41 0 top
U$57  [A10]  50.55,29.21 0 top
U$58  [A10]  54.1,29.21 0 bottom
U$59  [PWM01]  48.01,31.75 0 top
U$60  [PWM01]  54.23,31.75 0 bottom
U$61  [PWM10]  54.36,34.29 0 bottom
U$62  [Y1]  43.05,5.71 0 top
U$63  [Z2]  37.85,5.71 0 top
U$64  [#VE#0]  24.64,8.51 0 bottom
U$65  [MACHINE2]  38.99,23.24 0 bottom
U$66  [LEARNING3]  29.84,23.24 0 bottom
U$67  [EN22]  37.47,20.95 0 top
VE  25.4,8.51 0 bottom
VIN_LED  50.8,2.54 0 bottom

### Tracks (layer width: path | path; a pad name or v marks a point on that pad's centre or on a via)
1.8V  (via drill 0.3)
  Top 0.178: C23.1 TP7.P$1 9.27,50.8 | J7.10 21.61,50.4 20.86,51.15 9.62,51.15 9.27,50.8 | U3.5 9.21,50.74 9.27,50.8
  other vias: 7.62,50.8
3.3V  (via drill 0.3)
  Top 0.178: 18.67,43.69 22.1,43.69 | 22.1,43.69 v27.98,43.69 33.02,43.69 | U4.3 U4.2 U4.9 U4.10 36.73,12.18 | J7.4 18.61,43.75 18.67,43.69 | J7.11 22.11,43.7 22.1,43.69 | J11.VCC 42.62,46.41 42.29,46.74 34.04,46.74 33.02,45.72 33.02,43.69 | 33.02,43.69 C46.1 | 36.73,12.18 C29.1 C30.1 | 36.73,12.18 38.48,12.18 v38.48,13.46 | v47.5,5.75 47.5,5.8 | MEAS.2 MEAS.4 | JP1.2 v45.72,10.16 | J2.1 14.79,22.86 15.56,23.63 16.19,23.63 17.48,22.34 17.48,18.59 18.29,17.78 v27.66,17.78 29.11,17.78 30.44,19.11 30.44,19.77 31.62,20.95 EN1.2 | v9.27,40.51 9.21,40.57 9.21,45.21 | U3.1 9.21,45.21 | 18.67,43.69 15.24,43.69 14.73,43.69 14.22,43.69 12.7,45.21 | J4.74 28.43,29.32 v28.45,29.34 | D3.2 9.29,37.2 v9.27,37.21 | v34.92,15.24 35.15,15.47 39.18,15.47 C31.1 | EN2.2 36.42,21.61 v35.94,22.1 | 12.7,45.21 9.21,45.21 | C22.1 12.7,45.21
  Top 0.254: C3.1 13.97,5.8 | C4.1 15.49,5.8 | C5.1 17.02,5.8
  Top 0.305: J4.2 v28.56,11.32
  Top 0.559: 28.96,5.8 17.02,5.8 15.49,5.8 13.97,5.8 13.3,5.8 12.75,6.35 MEAS.4 | 28.96,5.8 47.5,5.8 50.39,5.8 52.23,7.65 52.23,8.89 52.75,9.41 J3.2 55.1,9.41 55.78,10.09 55.78,10.74 55.24,11.27 55.24,19.68 J14.2 | v28.56,11.32 28.96,10.92 28.96,5.8
  Bottom 0.178: v27.98,43.69 27.74,43.45 27.74,40.08 28.57,39.24 28.57,29.8 28.45,29.68 v28.45,29.34 | v9.27,40.51 v9.27,37.21 | 3V3_LED.2 42.66,3.92 44.49,5.75 45.76,5.75 | 45.76,5.75 v47.5,5.75 | 45.76,5.75 45.72,5.79 v45.72,10.16 | 34.92,13.46 v34.92,15.24 34.2,15.96 34.2,19.09 35.94,20.83 v35.94,22.1 | 34.92,13.46 34.92,12.7 33.66,11.43 28.67,11.43 v28.56,11.32 | v38.48,13.46 34.92,13.46
  Bottom 0.305: v28.56,11.32 28.56,12.38 28.6,12.43 28.6,14.01 27.66,14.95 v27.66,17.78 27.66,18.1 28.45,18.89 v28.45,29.34
3.3V_EN  (via drill 0.3)
  Top 0.178: v25.11,11.81 v25.12,11.82 J4.4
  Bottom 0.178: VE.1 25.81,11.11 v25.11,11.81
!BOOT!  (via drill 0.3)
  Top 0.178: v22.48,13.46 22.37,13.57 J4.11 | S2.4 v34.29,6.99 S2.3
  Bottom 0.178: v22.48,13.46 22.48,8.55 24.05,6.99 v34.29,6.99
!RESET!  (via drill 0.3)
  Top 0.178: v27.94,12.7 27.56,12.32 J4.6 | v17.78,8.89 19.68,6.99 S1.4 S1.3 27.56,6.99 27.94,7.37 v27.94,8.89 | J2.10 16.41,17.25 16.41,16.62 17.4,15.63 v17.4,14.61
  Bottom 0.178: v27.94,12.7 v27.94,8.89 | v17.4,14.61 17.4,14.02 16.29,12.91 16.29,9.87 17.27,8.89 v17.78,8.89 J9.1
A0  (via drill 0.3)
  Top 0.178: J8.1 52.51,24.57 40.9,24.57 40.55,24.92 v31.7,24.92 | J4.34 29.1,19.32 v29.21,19.43
  Bottom 0.178: v29.21,19.43 31.7,21.92 v31.7,24.92
A1  (via drill 0.3)
  Top 0.178: v30.86,24.92 31.1,25.16 31.45,25.51 40.46,25.51 41.05,24.93 50.33,24.93 J8.2 | J4.38 v29.21,20.32
  Bottom 0.178: v29.21,20.32 30.86,21.97 v30.86,24.92
CAMERA_D0  (via drill 0.3)
  Top 0.178: J7.14 23.61,49.65 v23.82,49.85 | J4.40 v21.73,20.82 v21.72,20.83
  Bottom 0.178: v23.82,49.85 23.84,49.83 23.84,47.93 24.41,47.36 24.41,41.61 20.78,37.98 20.78,26.3 21.34,25.74 21.34,22.25 21.75,21.84 21.75,21.34 21.72,21.31 v21.72,20.83
CAMERA_D1  (via drill 0.3)
  Top 0.178: v29.21,21.34 29.19,21.32 J4.42 | v18.55,42.15 29.22,42.15 v29.34,42.04 | J7.3 18.11,49.61 v18.16,49.66
  Bottom 0.178: v29.21,21.34 29.63,21.75 30.09,21.75 30.44,22.11 30.44,22.6 30.2,22.84 30.2,28.43 30.29,28.52 30.29,41.22 29.47,42.04 v29.34,42.04 | v18.55,42.15 18.87,42.47 18.87,47.99 18.16,48.71 v18.16,49.66
CAMERA_D2  (via drill 0.3)
  Top 0.178: v21.15,21.59 25.15,21.59 25.38,21.82 J4.44 | J7.9 21.11,48.61 v20.83,48.9
  Bottom 0.178: v20.83,48.9 23.34,46.38 23.34,42.18 19.23,38.07 19.23,23.27 20.19,22.31 20.44,22.31 v21.15,21.6 v21.15,21.59
CAMERA_D3  (via drill 0.3)
  Top 0.178: v29.84,22.35 29.81,22.32 J4.46 | v18.99,41.4 28.76,41.4 v28.78,41.38 | J7.5 19.11,48.62 v18.88,48.85
  Bottom 0.178: v29.84,22.35 29.84,28.58 29.93,28.67 29.93,40.77 29.33,41.38 v28.78,41.38 | v18.88,48.85 19.14,48.59 19.14,48.23 19.23,48.14 19.23,41.64 v18.99,41.4
CAMERA_D4  (via drill 0.3)
  Top 0.178: v20.23,23.11 20.52,22.82 J4.48 | J7.12 22.61,48.62 v22.34,48.89
  Bottom 0.178: v22.34,48.89 22.34,48.17 23.7,46.81 23.7,42.03 19.58,37.92 19.58,27.73 20.23,27.08 v20.23,23.11
CAMERA_D5  (via drill 0.3)
  Top 0.178: J7.20 26.61,50.1 v26.8,50.29 | v25.12,27.43 24.61,27.43 22.98,29.07 J4.73
  Bottom 0.178: v25.12,27.43 25.12,27.65 26.54,29.07 26.54,48.13 26.78,48.37 26.78,50.28 v26.8,50.29
CAMERA_D6  (via drill 0.3)
  Top 0.178: v22.99,28.09 22.51,28.57 J4.71 | J7.19 26.11,48.49 v25.83,48.77
  Bottom 0.178: v25.83,48.77 25.83,40.97 22.73,37.87 22.73,28.35 v22.99,28.09
CAMERA_D7  (via drill 0.3)
  Top 0.178: v20.18,27.97 20.08,28.07 J4.69 | J7.13 23.11,49.31 v23.01,49.4
  Bottom 0.178: v20.18,27.97 20.18,38.01 24.05,41.88 24.05,46.99 23.01,48.03 v23.01,49.4
CAMERA_HSYNC  (via drill 0.3)
  Top 0.178: v24.43,50.42 24.45,50.41 24.45,48.39 24.45,48.3 24.61,48.14 J7.16 | v21.37,26.54 20.85,27.07 J4.65
  Bottom 0.178: v24.43,50.42 24.45,50.41 24.45,48.21 24.77,47.89 24.77,41.47 21.61,38.32 21.61,26.78 v21.37,26.54
CAMERA_INT  (via drill 0.3)
  Top 0.178: v25.4,49.53 25.4,49.18 25.23,49.02 25.23,48.52 25.61,48.15 J7.18 | v22.61,16.26 24.04,14.82 J4.16
  Bottom 0.178: v25.4,49.53 25.4,49.18 25.23,49.02 25.23,48.42 25.48,48.18 25.48,41.17 22.33,38.02 22.33,25.25 22.57,25.01 22.57,16.29 v22.61,16.26
CAMERA_MCLK  (via drill 0.3)
  Top 0.178: v20.45,49.78 20.45,49.36 20.23,49.14 20.23,48.65 20.61,48.27 J7.8 | v24.51,25.5 25.19,24.82 J4.56
  Bottom 0.178: v24.51,25.5 24.51,27.67 26.19,29.34 26.19,48.28 26.43,48.52 26.43,49.34 26.12,49.65 26.12,50.74 25.85,51.02 23.78,51.02 22.55,49.78 v20.45,49.78
CAMERA_VSYNC  (via drill 0.3)
  Top 0.178: v16.49,27.03 16.51,27.03 16.97,26.57 J4.63 | v19.25,49.66 19.49,49.42 19.49,48.38 19.61,48.26 J7.6
  Bottom 0.178: v19.25,49.66 19.49,49.42 19.49,48.38 19.58,48.29 19.58,40.02 16.49,36.93 v16.49,27.03
D0/HEADER_!CS!  (via drill 0.3)
  Top 0.178: v29.84,13.08 29.61,13.32 J4.10 | J8.5 49.53,31.75 v34.29,31.75 33.53,30.99 32.38,30.99 31.62,31.75 31.62,35.43 30.99,36.07 3.05,36.07 J5.4
  Bottom 0.178: v29.84,13.08 29.84,17.84 31.41,19.41 33.19,19.41 34.04,20.26 34.04,22.12 33.01,23.16 33.01,30.47 v34.29,31.75
D1/CAMERA_TRIG  (via drill 0.3)
  Top 0.178: v28.32,15.22 28.22,15.32 J4.18 | v19.98,50.5 19.98,50.16 19.85,50.03 19.85,48.53 20.11,48.27 J7.7 | J8.6 47.35,32.11 34.78,32.11 34.54,32.35 33.06,32.35 33.02,32.38 | v20.18,42.93 29.34,42.93 33.02,39.24 33.02,32.38 | 33.02,32.38 v33.02,31.75
  Bottom 0.178: v28.32,15.22 28.32,16.82 31.39,19.89 33.04,19.89 33.69,20.54 33.69,21.85 32.65,22.89 32.65,31.38 v33.02,31.75 | v19.98,50.5 19.98,50.16 19.85,50.03 19.85,48.53 20.18,48.2 v20.18,42.93
GND  (via drill 0.3)
  Top 0.178: 33.02,20.07 33.07,20.02 | E2.8 E2.9 E2.3 E2.7 | E2.8 E2.7 | E2.7 37.77,17.36 C31.2 | E1.2 32.37,18.08 | E1.8 E1.6 E1.3 E1.7 32.64,15.75 v31.75,15.75 | E2.8 36.83,18.03 36.54,18.32 E2.2 | J7.2 17.61,48.56 v17.4,48.77 | J7.15 24.11,46.21 23.75,45.85 v22.73,45.85
  Top 0.559: J1.GND 7.46,13.38 R2.1 | J1.GND2 7.46,6.93 R3.1
  other vias: 12.7,7.87 10.16,10.16 8.89,10.16 11.43,10.16 7.75,10.16 7.24,14.86 12.19,15.11 11.81,17.78 7.75,5.59 11.05,7.87 17.4,10.92 20.19,12.57 24.89,19.81 20.19,21.72 20.19,20.83 17.65,45.85 12.7,27.94 29.46,46.61 10.16,48.26 13.97,49.53 7.62,46.23 44.83,43.69 39.37,22.48 36.83,22.61 34.67,9.78 37.47,9.27 53.98,7.37 20.19,11.18 16.51,14.22 17.27,29.59 20.32,19.05 31.75,41.78 15.75,9.02 24.13,2.54 34.29,2.54 35.69,16.13
  pour Bottom (isolate 0.178): 0,52.07 58.42,52.07 58.42,0 0,0
  pour Top (isolate 0.178, rank 3): 0,52.07 58.42,52.07 58.42,0 0,0
I2C_SCL  (via drill 0.3)
  Top 0.178: v53.85,12.32 53.59,12.06 J3.4 50.82,11.41 50.38,11.85 R4.1 50.38,13.37 49.91,13.84 47.92,13.84 46.98,12.9 40.77,12.9 39.36,14.32 33.53,14.32 | J7.21 27.11,49.39 v27.38,49.66 | v24.13,14.22 24.23,14.32 J4.14 33.53,14.32 | 33.53,14.32 33.54,14.31 U4.1
  Bottom 0.178: v53.85,12.32 53.89,12.28 53.89,10.29 54.36,9.82 56.63,9.82 57.15,10.33 J14.4 | v27.38,49.66 27.14,49.42 27.14,48.23 26.9,47.98 26.9,27.05 24.76,24.91 24.65,24.91 23.24,23.5 23.24,15.2 23.33,15.11 23.33,15.02 v24.13,14.22
I2C_SDA  (via drill 0.3)
  Top 0.178: v54.99,10.41 v54.98,10.41 J3.3 52.06,10.41 51.69,10.03 51.69,7.87 51.44,7.62 R1.1 50.42,7.58 50.42,6.6 50.16,6.35 43.69,6.35 42.16,7.87 34.8,7.87 33.54,9.13 U4.4 33.15,10.68 32.89,10.93 32.89,12.57 31.65,13.82 J4.12 25.12,13.82 v24.89,13.59 | J7.22 27.61,48.7 v27.81,48.9
  Bottom 0.178: v54.99,10.41 54.99,16.89 J14.3 | v27.81,48.9 27.5,48.59 27.5,48.08 27.25,47.84 27.25,26.36 24,23.11 24,15.19 24.73,14.47 24.73,13.75 v24.89,13.59
I2S_SCK/PDM_CLK  (via drill 0.3)
  Top 0.178: J4.50 33.88,23.32 34.67,22.52 34.67,18.03 | v38.86,18.92 38.26,18.32 E2.4 | v34.8,17.14 34.67,17.27 34.67,18.03 | E1.4 34.62,18.08 34.67,18.03
  Bottom 0.178: v34.8,17.14 35.18,17.14 36.7,18.67 38.61,18.67 v38.86,18.92
I2S_SD/CAMERA_PCLK  (via drill 0.3)
  Top 0.178: v37.34,24.26 37.27,24.32 J4.54 22,24.32 v21.93,24.26 | v25.4,50.37 25.16,50.13 25.15,50.13 24.8,49.78 24.8,48.45 25.11,48.14 J7.17 | E2.6 v36.83,19.81
  Bottom 0.178: v25.4,50.37 25.16,50.13 25.15,50.13 24.8,49.78 24.8,48.35 25.12,48.04 25.12,41.32 21.97,38.17 21.97,24.3 v21.93,24.26 | v36.83,19.81 36.83,21.76 37.43,22.36 37.43,24.17 v37.34,24.26
I2S_WS/PDM_DAT
  Top 0.178: J4.52 34.22,23.82 35.05,22.99 35.05,19.14 | 35.05,19.14 E2.1 | 35.05,19.14 35.05,17.73 35.4,17.39 35.4,16.81 33.57,14.99 31.37,14.99 30.99,15.37 30.99,18.73 31.34,19.08 E1.1
N$1  (via drill 0.3)
  Top 0.178: R6.2 49.95,4.61 50.42,5.08 v51.56,5.08
  Bottom 0.178: VIN_LED.1 51.32,4.84 v51.56,5.08
N$2
  Top 0.178: R4.2 48.68,12.03 49.51,11.2 JP1.3
N$3
  Top 0.178: JP1.1 49.53,8.47 R1.2
N$4
  Top 0.178: E1.5 33.92,19.67 33.54,20.05 EN1.1
N$5
  Top 0.178: E2.5 37.73,20.18 37.24,20.68 EN2.1
N$6  (via drill 0.38)
  Top 0.178: R11.2 43.81,3.81 v43.69,3.94
  Bottom 0.178: v43.69,3.94 43.69,2.55 3V3_LED.1
N$7
  Top 0.178: R11.1 47.84,2.57 D2.A
N$8
  Top 0.178: R6.1 51.65,2.57 D4.A
N$10
  Top 0.178: J1.A5 7.18,11.41 R2.2
N$11
  Top 0.178: J1.B5 7.56,8.41 R3.2
N$12  (via drill 0.3)
  Top 0.178: U5.5 11.13,12.28 11.43,12.57 12.7,12.57 | v16.89,12.67 16.8,12.57 12.7,12.57 | D1.C 13,11.31 R5.1 12.7,12.57
  Bottom 0.178: VE.2 23.62,8.51 23.08,9.05 23.08,13.71 22.73,14.06 20.99,14.06 20.95,14.1 18.32,14.1 v16.89,12.67
N$14
  Top 0.178: BT1.+ 10.67,31.66 R8.1 10.28,32.05 D6.A
PWM0  (via drill 0.3)
  Top 0.178: v29.08,18.59 28.86,18.82 J4.32 | v31.75,29.21 52.07,29.21 J8.3
  Bottom 0.178: v29.08,18.59 29.32,18.83 29.46,18.83 32.3,21.67 32.3,25.16 31.75,25.71 v31.75,29.21
PWM1/CAM_VDD  (via drill 0.3)
  Top 0.178: v24.77,22.22 24.52,22.46 20.04,22.46 19.93,22.57 J4.47 | J8.4 50.37,30.05 v27.98,30.05 27.98,33.24 26.67,34.54 v14.22,34.54 | U3.3 11.11,45.91 v11.05,45.85
  Bottom 0.178: v24.77,22.22 25.68,23.14 27.07,23.14 27.74,23.81 27.74,29.81 v27.98,30.05 | v11.05,45.85 14.22,42.67 v14.22,34.54
RTC_3V
  Top 0.178: R8.2 12.58,32.05 D6.C | J4.72 23.73,28.82 23.12,29.43 22.52,29.43 21.59,30.35 21.59,31.75 19.81,33.53 D6.C | D6.C 12.19,33.53 11.43,34.29 D3.3
RX1  (via drill 0.3)
  Top 0.178: v20.45,15.62 20.4,15.57 J4.19
  Bottom 0.178: v20.45,15.62 14.81,15.62 3.77,26.67 J6.2
SDIO_DAT1  (via drill 0.3)
  Top 0.178: v47.12,27.43 46.81,27.13 39.12,27.13 38.93,27.32 J4.66 | J11.DAT1 47.02,43.28 v47.12,43.18
  Bottom 0.178: v47.12,27.43 v47.12,43.18
SDIO_DAT2  (via drill 0.3)
  Top 0.178: v39.37,27.72 39.27,27.82 J4.68 | J11.DAT2 39.32,42.59 v39.37,42.55
  Bottom 0.178: v39.37,42.55 v39.37,27.72
SPI_!CS!/SDIO_DAT3  (via drill 0.3)
  Top 0.178: v40.39,28.32 v40.38,28.32 J4.70 | J11.CS/DAT3 40.42,43.09 v40.39,43.05
  Bottom 0.178: v40.39,28.32 v40.39,43.05
SPI_SCK  (via drill 0.3)
  Top 0.178: v43.69,25.53 43.64,25.58 40.9,25.58 40.61,25.87 31.3,25.87 31.25,25.82 J4.60 | J11.SCLK 43.72,43.09 v43.69,43.05 | J5.1 6.98,41.91 9.01,39.88 31.24,39.88 v31.75,39.37
  Bottom 0.178: v43.69,25.53 v43.69,43.05 42.17,43.05 41.54,43.69 39.62,43.69 35.3,39.37 v31.75,39.37
SPI_SDI  (via drill 0.3)
  Top 0.178: v45.97,26.53 45.73,26.77 38.98,26.77 38.93,26.82 J4.64 26.39,26.84 24.88,26.84 24.79,26.92 v23.91,26.92 | J11.DO/DAT0 45.92,43.23 v45.97,43.18 | v25.59,38.74 25.29,38.74 24.85,38.3 2.74,38.3 J5.3
  Bottom 0.178: v45.97,43.18 v45.97,26.53 | v25.59,38.74 25.83,38.5 25.83,29.49 24.16,27.82 24.16,27.16 v23.91,26.92
SPI_SDO  (via drill 0.3)
  Top 0.178: v41.15,26.17 41,26.32 J4.62 23.53,26.32 v23.43,26.22 | J11.DI/CMD v41.53,42.8 | J5.2 24.13,39.37 v24.6,38.9
  Bottom 0.178: v41.53,42.8 41.15,42.42 v41.15,26.17 | v23.43,26.22 23.43,26.57 23.32,26.68 23.32,27.48 25.48,29.64 25.48,38.01 24.99,38.49 24.99,38.51 v24.6,38.9
SWDCK
  Top 0.178: J2.4 16.76,20.7 16.76,16.76 17.46,16.07 J4.21
SWDIO
  Top 0.178: J2.2 17.12,21.61 17.12,17.04 17.59,16.57 J4.23
TX1  (via drill 0.3)
  Top 0.178: v21.46,14.82 21.26,15.02 20.2,15.02 20.15,15.07 J4.17
  Bottom 0.178: v21.46,14.82 21.04,15.24 21.04,15.87 20.69,16.22 20.2,16.22 20.11,16.13 14.81,16.13 1.73,29.21 J6.1
USB_D+  (via drill 0.3)
  Top 0.178: J1.B6 5.2,9.41 5.08,9.53 5.08,9.78 | 5.08,9.78 5.08,10.29 5.2,10.41 J1.A6 | v15.62,11.6 15.65,11.57 J4.3 | v4.75,9.78 5.08,9.78
  Bottom 0.178: v15.62,11.6 15.62,11.47 15.49,11.34 6.31,11.34 v4.75,9.78
USB_D-  (via drill 0.3)
  Top 0.178: J1.B7 6.1,10.91 | 6.1,10.91 6.87,10.91 6.99,10.79 6.99,10.03 6.86,9.91 J1.A7 | v4.85,10.9 6.09,10.9 6.1,10.91 | v13.72,11.94 13.97,12.2 15.99,12.2 16.12,12.07 J4.5
  Bottom 0.178: v13.72,11.94 5.89,11.94 v4.85,10.9
V_USB
  Top 0.305: J1.VBUS1 5.39,12.61 5.18,12.39 4.14,12.39 3.81,12.06 3.81,8.26 4.14,7.92 5.18,7.92 5.39,7.71 J1.VBUS2
  Top 0.559: BYP.1 2.92,20.32 2.31,19.71 F2.1 2.31,15.97 2.77,15.51 2.77,12.73 3.1,12.39 4.14,12.39
VIN  (via drill 0.3)
  Top 0.178: v21.59,12.97 21.39,13.17 19.95,13.17 19.85,13.07 J4.9 | R5.2 13.42,10.03 v17.4,10.03
  Top 0.305: 9.31,13.08 9.31,13.09 13.72,13.09 | R10.2 13.72,13.09 | 13.72,13.09 16.38,13.09 16.62,13.33 17.28,13.33 17.54,13.07 J4.9
  Top 0.559: BYP.2 4.95,20.32 5.31,19.96 F2.2 C2.+ 7.49,16.17 8.17,15.49 C1.1 C13.1 9.31,13.08
  Bottom 0.178: v17.4,10.03 16.76,10.67 16.76,11.43 18.5,13.17 21.39,13.17 v21.59,12.97 22.12,12.44 22.12,8.41 23.9,6.63 24.61,6.63 24.85,6.39 37.05,6.39 40.51,2.92 40.51,2.16 42.16,0.51 46.86,0.51 48.9,2.54 VIN_LED.2
  pour Top (isolate 0.178, rank 2): 10.16,11.05 8.38,11.05 8.38,14.35 10.16,14.35
VIN/3
  Top 0.178: R9.2 R10.1 13.72,23.75 13.95,23.98 16.34,23.98 17.25,23.07 J4.49
VREG_3.3V
  Top 0.178: MEAS.1 MEAS.3
  pour Top (isolate 0.305): 8.38,9.27 8.38,6.35 10.16,6.35 10.16,9.27

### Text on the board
Bottom: v12
tPlace: + | -
tDocu: N. Seidle

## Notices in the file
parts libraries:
SparkFun-Aesthetics: Licensing: Creative Commons ShareAlike 4.0 International - https://creativecommons.org/licenses/by-sa/4.0
SparkFun-Aesthetics: Released under the Creative Commons Attribution Share-Alike 4.0 License
SparkFun-Aesthetics: https://creativecommons.org/licenses/by-sa/4.0
